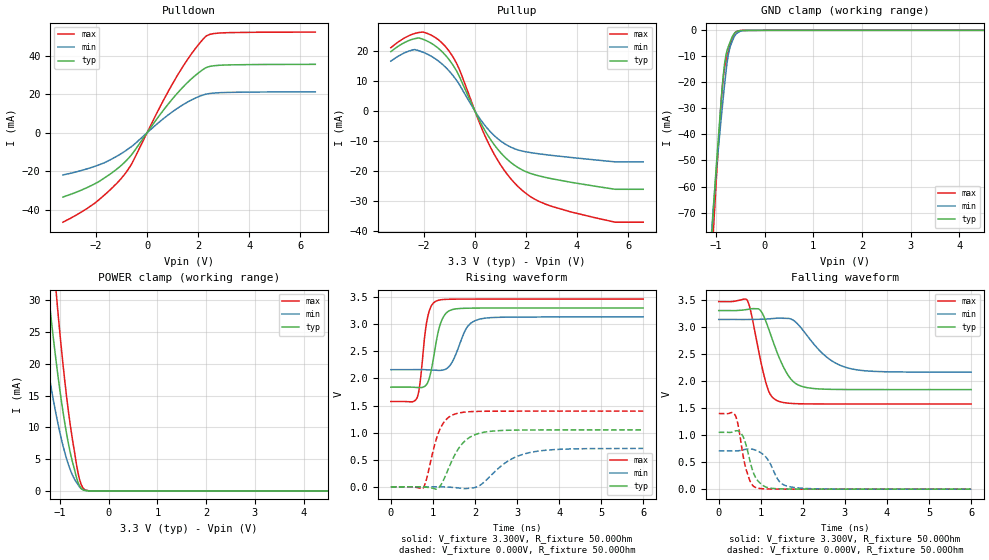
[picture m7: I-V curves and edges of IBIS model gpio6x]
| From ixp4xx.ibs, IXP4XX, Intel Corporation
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[Model]   gpio6x
Model_type   I/O
Vinl = 800.000mV
Vinh = 2.000V
Vmeas = 1.500V
Cref = 0.000F
|   typ   min   max
C_comp   3.000pF   2.700pF   3.300pF
[Voltage Range]   3.300V   3.135V   3.465V
[Temperature Range]   25.0   110.0   -40.0
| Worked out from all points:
|   slope of the pulldown table from 0 to 0.495 V, typ, clamps not added: 54 ohm
|   slope of the pullup table from 0 to 0.495 V, typ, clamps not added: 62.1 ohm
|   GND clamp passes 1 mA (typ) near -0.61 V on its own axis
|   POWER clamp passes 1 mA (typ) near -0.61 V on its own axis
|   falling waveform, V_fixture 3.300V, R_fixture 50.00Ohm: 20-80 % time 462ps typ, 720ps min, 312ps max; typ from 3.3 V to 1.84 V
|   rising waveform, V_fixture 3.300V, R_fixture 50.00Ohm: 20-80 % time 223ps typ, 315ps min, 165ps max; typ from 1.84 V to 3.3 V
|   rising waveform, V_fixture 0.000V, R_fixture 50.00Ohm: 20-80 % time 452ps typ, 729ps min, 311ps max; typ from 0 V to 1.05 V
|   falling waveform, V_fixture 0.000V, R_fixture 50.00Ohm: 20-80 % time 240ps typ, 295ps min, 210ps max; typ from 1.05 V to 0 V
[Pulldown]
|   Voltage   I(typ)   I(min)   I(max)
-3.3V     -33.43mA   -21.96mA   -46.5mA
-2.07V    -26.7mA    -17.56mA   -36.8mA
-1.4V     -21.03mA   -13.76mA   -29.11mA
-905mV    -15.67mA   -9.933mA   -22.05mA
-580mV    -10.96mA   -6.892mA   -15.58mA
510mV     9.441mA    5.9mA      13.54mA
1.13V     19.68mA    12.16mA    28.46mA
1.73V     27.91mA    16.97mA    40.82mA
2.3V      33.74mA    20.02mA    50.07mA
2.6V      34.79mA    20.61mA    51.52mA
3.115V    35.23mA    20.95mA    52mA
6.595V    35.56mA    21.26mA    52.32mA
[GND Clamp]
|   Voltage   I(typ)   I(min)   I(max)
-3.3V     -1.979A    -1.804A    -2.12A
-1.11V    -87.92mA   -83.88mA   -99.37mA
-1.065V   -73.04mA   -71.51mA   -82.02mA
-1.05V    -68.59mA   -67.61mA   -76.83mA
-985mV    -50.68mA   -52.6mA    -55.53mA
-900mV    -29.25mA   -35.73mA   -29.78mA
-850mV    -17.83mA   -26.3mA    -18.42mA
-790mV    -9.3mA     -15.6mA    -11.42mA
-745mV    -6.333mA   -9.483mA   -8.213mA
-670mV    -2.684mA   -4.492mA   -3.293mA
-575mV    -476.6uA   -1.211mA   -444.8uA
6.595V    0A         0A         0A
[Pullup]
|   Voltage   I(typ)   I(min)   I(max)
-3.3V     19.87mA    16.69mA    21.19mA
-2.585V   23.59mA    20.07mA    25.21mA
-2.2V     24.43mA    20.17mA    26.26mA
-1.745V   22.81mA    18.47mA    25.49mA
-1.255V   19.55mA    15.47mA    22.45mA
-700mV    13.07mA    10.01mA    15.57mA
190mV     -3.355mA   -2.494mA   -4.218mA
665mV     -10.17mA   -7.425mA   -13mA
1.4V      -17.1mA    -12mA      -22.54mA
2.11V     -20.6mA    -13.76mA   -28.17mA
4.685V    -25.04mA   -16.27mA   -35.56mA
6.595V    -26.1mA    -16.94mA   -37.09mA
[POWER Clamp]
|   Voltage   I(typ)   I(min)   I(max)
-3.3V     262.4mA    183.1mA    340.6mA
-1.46V    48.9mA     30.49mA    70.7mA
-1.24V    31.26mA    18.92mA    46.56mA
-1.085V   20.72mA    12.21mA    31.79mA
-1.065V   19.49mA    11.44mA    30.04mA
-930mV    12.02mA    6.852mA    19.28mA
-855mV    8.57mA     4.804mA    14.2mA
-785mV    5.873mA    3.236mA    10.14mA
-630mV    1.332mA    997.1uA    2.826mA
-565mV    412.5uA    348.1uA    1.013mA
-515mV    136.2uA    138.7uA    344.2uA
6.595V    0A         0A         0A
[Ramp]
R_load = 50.00Ohm
|   typ   min   max
dV/dt_r   630.059mV/451.534ps 424.896mV/728.064ps 837.767mV/310.207ps
dV/dt_f   876.153mV/462.057ps 583.761mV/718.826ps   1.135V/312.108ps
[Falling Waveform]
V_fixture = 3.300V
V_fixture_min = 3.135V
V_fixture_max = 3.465V
R_fixture = 50.00Ohm
|   Time   V(typ)   V(min)   V(max)
0s        3.3V       3.135V     3.465V
680ps     3.32V      3.134V     3.486V
970ps     3.318V     3.138V     2.471V
1.14ns    3.061V     3.143V     1.918V
1.41ns    2.483V     3.16V      1.628V
1.65ns    2.104V     3.155V     1.589V
1.89ns    1.925V     3.04V      1.578V
2.5ns     1.848V     2.483V     1.574V
3.08ns    1.841V     2.237V     1.574V
6ns       1.84V      2.162V     1.574V
[Rising Waveform]
V_fixture = 3.300V
V_fixture_min = 3.135V
V_fixture_max = 3.465V
R_fixture = 50.00Ohm
|   Time   V(typ)   V(min)   V(max)
0s        1.84V      2.162V     1.574V
620ps     1.834V     2.163V     1.638V
690ps     1.831V     2.164V     1.891V
870ps     1.913V     2.159V     3.11V
1.09ns    2.721V     2.15V      3.432V
1.2ns     3.053V     2.15V      3.452V
1.36ns    3.235V     2.201V     3.461V
1.8ns     3.296V     2.929V     3.465V
2.09ns    3.299V     3.09V      3.465V
6ns       3.3V       3.135V     3.465V
[Rising Waveform]
V_fixture = 0.000V
V_fixture_min = 0.000V
V_fixture_max = 0.000V
R_fixture = 50.00Ohm
|   Time   V(typ)   V(min)   V(max)
0s        68.08nV    533.2nV    41.51nV
760ps     -3.07mV    267.4uV    -31.48mV
1.17ns    11.11mV    -539uV     1.066V
1.33ns    261.1mV    -4.836mV   1.253V
1.55ns    629.8mV    -16.2mV    1.349V
1.79ns    865.3mV    -32.78mV   1.381V
2.07ns    980mV      5.846mV    1.392V
2.78ns    1.043V     471.8mV    1.396V
3.35ns    1.049V     639.2mV    1.396V
6ns       1.05V      708.2mV    1.396V
[Falling Waveform]
V_fixture = 0.000V
V_fixture_min = 0.000V
V_fixture_max = 0.000V
R_fixture = 50.00Ohm
|   Time   V(typ)   V(min)   V(max)
0s        1.05V      708.2mV    1.396V
390ps     1.075V     705.9mV    1.367V
540ps     1.023V     720.6mV    806.2mV
650ps     814.4mV    737.8mV    369.4mV
770ps     438.4mV    740.6mV    109.5mV
900ps     185.3mV    714.1mV    25.15mV
1.16ns    30.14mV    554.5mV    4.15mV
1.45ns    6.545mV    135.5mV    950.9uV
1.69ns    2.534mV    44.85mV    296.6uV
6ns       68.08nV    533.2nV    41.51nV
